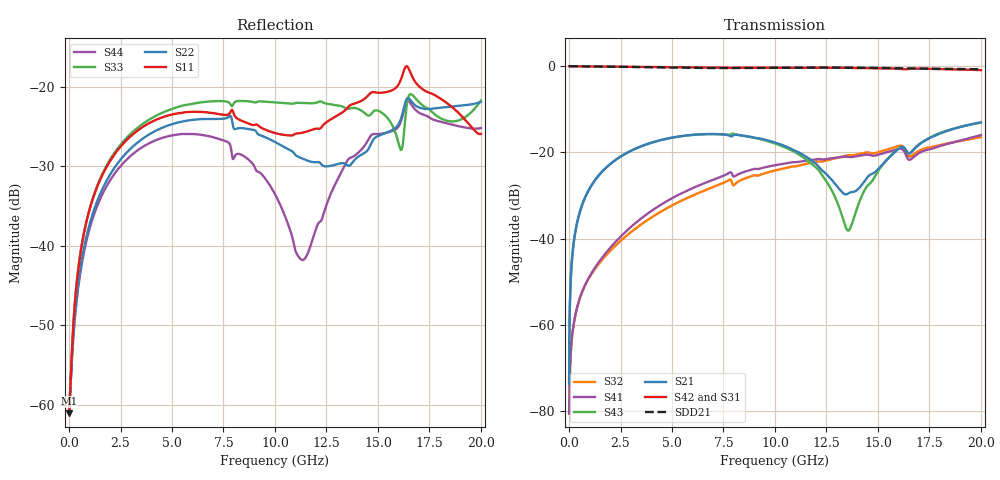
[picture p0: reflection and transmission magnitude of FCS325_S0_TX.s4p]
!Generated from:
! 1
! 2
! 3
! 4
!PowerSI Version: 17.0.2.03131.86335  002
!Computer Host Name: W764D-PINDIS
!TouchstoneFormatFlag = 1
! GNDNET
! NETSLIST
!User Comments:
!  Touchstone file from project M5P200_FCS325_111116_1100_GW_0705_85Ohm_111717
!  Exported from HFSS 3D Layout Design 2017.2.0
!  Port[1] = BGA.D20.SERDES_0_TX0_N
!  Port[2] = BGA.D21.SERDES_0_TX0_P
!  Port[3] = DIE.410.SERDES_0_TX0_N
!  Port[4] = DIE.411.SERDES_0_TX0_P
!  freq  S11mag  S11ang  S12mag
!  S12ang  S13mag  S13ang  S1
!  4mag  S14ang
!  S21mag  S21ang  S22mag
!  S22ang  S23mag  S23ang  S2
!  4mag  S24ang
!  S31mag  S31ang  S32mag
!  S32ang  S33mag  S33ang  S3
!  4mag  S34ang
!  S41mag  S41ang  S42mag
!  S42ang  S43mag  S43ang  S4
!  4mag  S44ang
#	Hz	S	RI	R	50
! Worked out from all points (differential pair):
!   4999 points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, 4.001 MHz to 20 GHz, reference 50 ohm
!   strongest paths, dB at 4.001 MHz, 5.001 GHz, 10 GHz, 15 GHz, 20 GHz:
!     S42: 0.0, -0.3, -0.4, -0.5, -0.9
!     S31: 0.0, -0.3, -0.4, -0.5, -1.0
!     S21: -73.7, -16.6, -17.7, -23.9, -13.0
!     S43: -73.7, -16.6, -17.9, -24.4, -13.1
!     S41: -80.5, -30.6, -23.0, -20.6, -16.0
!     S32: -80.5, -32.3, -24.2, -20.0, -16.4
!   taken as a pair (ports 2,1 in; 4,3 out), SDD21 dB: 0.0, -0.4, -0.4, -0.4, -0.7
!   lowest |S11| = -61.1 dB at 4.001 MHz (marker M1), VSWR 1.00, Z = 50.1 + j0.00458 ohm
!   |S11| at or under -10 dB: start of sweep to end of sweep
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4000800  0.00088 4.58e-05  8.61e-05 0.000189  0.9991 -0.00105  -8.42e-05 -4.31e-05
         8.61e-05 0.000189  0.00089 6.67e-05  -8.42e-05 -4.31e-05  0.9991 -0.00105
         0.9991 -0.00105  -8.42e-05 -4.31e-05  0.00088 4.6e-05  8.61e-05 0.000189
         -8.42e-05 -4.31e-05  0.9991 -0.00105  8.61e-05 0.000189  0.00089 6.7e-05
1.680336e8  0.00198 -0.0016  0.000596 0.00671  0.9968 -0.0401  -0.000292 -0.00076
            0.000596 0.00671  0.00209 -0.000877  -0.000298 -0.000759  0.9968 -0.0397
            0.9968 -0.0401  -0.000298 -0.000759  0.00202 -0.00157  0.0006 0.00671
            -0.000292 -0.00076  0.9968 -0.0397  0.0006 0.00671  0.00205 -0.000852
5.481096e8  0.00256 -0.00845  0.00326 0.0211  0.987 -0.1262  -0.000544 -0.00205
            0.00326 0.0211  0.00339 -0.00627  -0.000615 -0.00203  0.9871 -0.1249
            0.987 -0.1262  -0.000615 -0.00203  0.00289 -0.00847  0.0034 0.021
            -0.000544 -0.00205  0.9871 -0.1249  0.0034 0.021  0.00297 -0.00606
2.828566e9  -0.026 -0.0388  0.0581 0.0805  0.7882 -0.5842  -0.00374 -0.012
            0.0581 0.0805  -0.0108 -0.0374  -0.0041 -0.0102  0.7926 -0.5788
            0.7882 -0.5842  -0.0041 -0.0102  -0.0151 -0.0459  0.0614 0.0781
            -0.00374 -0.012  0.7926 -0.5788  0.0614 0.0781  -0.0168 -0.0309
1.0018e10  -0.00191 0.0512  0.1186 -0.0531  -0.566 -0.7714  -0.057 0.0426
           0.1186 -0.0531  -0.0404 -0.0197  -0.0555 0.0271  -0.5469 -0.7878
           -0.566 -0.7714  -0.0555 0.0271  -0.0679 -0.0421  0.0945 -0.0838
           -0.057 0.0426  -0.5469 -0.7878  0.0945 -0.0838  -0.0136 0.0159
1.356271e10  0.0728 -0.0178  0.0333 0.00407  -0.9394 -0.1349  0.000191 0.0885
             0.0333 0.00407  -0.0119 -0.0296  -0.0197 0.0905  -0.9374 -0.1727
             -0.9394 -0.1349  -0.0197 0.0905  -0.063 -0.0365  -0.012 -0.00322
             0.000191 0.0885  -0.9374 -0.1727  -0.012 -0.00322  0.0193 -0.0293
2e10  0.00256 -0.0505  0.2121 0.0691  -0.2257 0.8631  0.1549 0.0353
      0.2121 0.0691  -0.00861 -0.0801  0.1472 0.0325  -0.3013 0.8471
      -0.2257 0.8631  0.1472 0.0325  -0.00718 -0.0818  0.2192 0.0305
      0.1549 0.0353  -0.3013 0.8471  0.2192 0.0305  -0.0207 -0.0511
